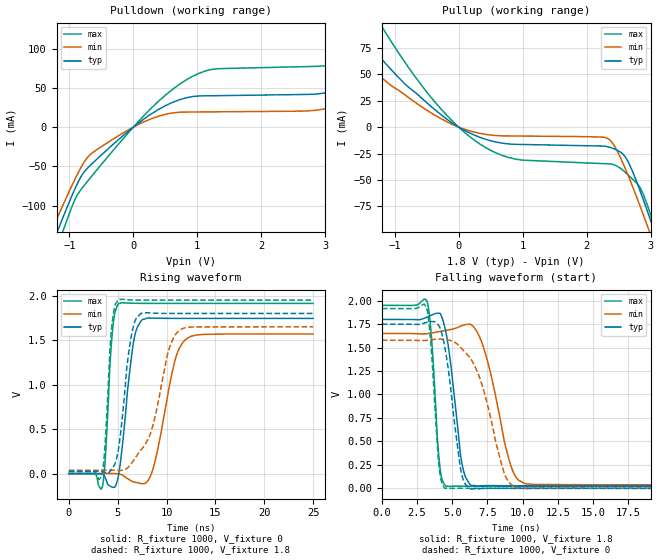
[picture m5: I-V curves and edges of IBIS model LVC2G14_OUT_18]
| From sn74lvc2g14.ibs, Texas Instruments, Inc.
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[Model]   LVC2G14_OUT_18
Model_type  Output
Vref =   0
Rref =   1000
Cref =   30p
Vmeas =   0.9
| variable   typ   min   max
C_comp   9.80pF   6.40pF   16.42pF
| C_pullup   9.15pF   6.40pF   10.43pF
| C_pulldown   10.45pF   6.59pF   16.42pF
[Temperature Range]   40   100   -40
| Ambient temperature   25   85   -40
[Voltage range]   1.8   1.65   1.95
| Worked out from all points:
|   slope of the pulldown table from 0 to 0.27 V, typ, clamps not added: 16.6 ohm
|   slope of the pullup table from 0 to 0.27 V, typ, clamps not added: 33 ohm
|   rising waveform, R_fixture 1000, V_fixture 0: 20-80 % time 995ps typ, 1.65ns min, 567ps max; typ from 0 V to 1.74 V
|   falling waveform, R_fixture 1000, V_fixture 1.8: 20-80 % time 780ps typ, 1.38ns min, 461ps max; typ from 1.8 V to 0.027 V
|   rising waveform, R_fixture 1000, V_fixture 1.8: 20-80 % time 1.02ns typ, 2.1ns min, 565ps max; typ from 0.027 V to 1.8 V
|   falling waveform, R_fixture 1000, V_fixture 0: 20-80 % time 868ps typ, 1.68ns min, 494ps max; typ from 1.75 V to 0 V
[Pulldown]
| LVC2G14_OUT_18
|   Voltage   I(typ)   I(min)   I(max)
-5.5V     -1.024A    -932.8mA   -1.143A
-1.25V    -145.7mA   -126.9mA   -167.2mA
-1.105V   -116mA     -100.2mA   -133.6mA
-650mV    -46.91mA   -33.3mA    -62.35mA
825mV     37.35mA    19.19mA    60.06mA
3.115V    45.49mA    25.17mA    79.66mA
3.755V    64.52mA    35.93mA    102.7mA
4.19V     79.14mA    21.53mA    128.2mA
4.47V     45.47mA    21.68mA    146.2mA
4.725V    44.49mA    21.83mA    131.7mA
5.01V     44.71mA    22mA       83.05mA
11V       50.72mA    25.33mA    92.94mA
[Pullup]
| LVC2G14_OUT_18
|   Voltage   I(typ)   I(min)   I(max)
-5.5V     449.7mA    254mA      638.5mA
-2.225V   143.3mA    107.6mA    207.3mA
-1.755V   105.1mA    78.04mA    153.5mA
-1.195V   63.95mA    46.44mA    94.81mA
-375mV    16.75mA    11.48mA    24.15mA
420mV     -11.47mA   -6.842mA   -19.31mA
2.34V     -18.76mA   -11.2mA    -34.79mA
2.645V    -32.43mA   -45.25mA   -45.19mA
2.84V     -61.19mA   -75.65mA   -57.82mA
2.99V     -86.8mA    -100.4mA   -81.09mA
3.08V     -102.8mA   -115.6mA   -97.77mA
11V       -1.709A    -1.61A     -1.847A
[Ramp]
| LVC2G14_OUT_18
| variable   typ   min   max
dV/dt_r   1.14/1.10E-09   1.01/1.80E-09   1.26/6.47E-10
dV/dt_f   1.10/8.47E-10   1.03/1.54E-09   1.20/5.07E-10
R_load = 1000
[Rising Waveform]
| LVC2G14_OUT_18
R_fixture =   1000
C_fixture =   0
L_fixture =   0
V_fixture =   0
V_fixture_min = 0
V_fixture_max = 0
|   Time   V(typ)   V(min)   V(max)
0s        112.7pV    7.663nV    3.037nV
3.43ns    -5.773mV   562.7uV    -148.1mV
4.45ns    -152.6mV   1.042mV    1.576V
5.115ns   -2.543mV   -3.276mV   1.911V
6.58ns    1.45V      -91.2mV    1.915V
7.51ns    1.729V     -113.8mV   1.913V
8.635ns   1.748V     59.81mV    1.913V
10.87ns   1.745V     1.273V     1.913V
11.9ns    1.744V     1.502V     1.913V
24.99ns   1.744V     1.569V     1.913V
[Falling Waveform]
| LVC2G14_OUT_18
R_fixture =   1000
C_fixture =   0
L_fixture =   0
V_fixture =   1.8
V_fixture_min = 1.65
V_fixture_max = 1.95
|   Time   V(typ)   V(min)   V(max)
0s        1.8V       1.65V      1.95V
3.225ns   1.826V     1.648V     1.988V
3.54ns    1.846V     1.656V     1.578V
4.075ns   1.867V     1.671V     293.4mV
4.54ns    1.668V     1.683V     22.36mV
5.625ns   317.2mV    1.731V     22.78mV
6.35ns    30.97mV    1.743V     21.2mV
7.295ns   27.96mV    1.464V     20.94mV
9.76ns    27.2mV     80.73mV    21.09mV
24.99ns   26.98mV    37.16mV    21.09mV
[Rising Waveform]
| LVC2G14_OUT_18
R_fixture =   1000
C_fixture =   0
L_fixture =   0
V_fixture =   1.8
V_fixture_min = 1.65
V_fixture_max = 1.95
|   Time   V(typ)   V(min)   V(max)
0s        26.95mV    37.1mV     21.07mV
3.365ns   24.61mV    37.5mV     -21.4mV
3.7ns     12.05mV    37.6mV     297.1mV
4.39ns    51.13mV    37.65mV    1.641V
5.125ns   303.9mV    35.74mV    1.958V
6.305ns   1.486V     98.9mV     1.952V
7.365ns   1.798V     262.7mV    1.95V
10.32ns   1.8V       1.421V     1.95V
11.41ns   1.8V       1.617V     1.95V
24.99ns   1.8V       1.65V      1.95V
[Falling Waveform]
| LVC2G14_OUT_18
R_fixture =   1000
C_fixture =   0
L_fixture =   0
V_fixture =   0
V_fixture_min = 0
V_fixture_max = 0
|   Time   V(typ)   V(min)   V(max)
0s        1.749V     1.578V     1.916V
3.185ns   1.769V     1.577V     1.914V
3.5ns     1.776V     1.584V     1.504V
4.035ns   1.734V     1.591V     267.6mV
4.485ns   1.492V     1.587V     -778.4uV
5.58ns    212.4mV    1.504V     1.161mV
6.295ns   -4.956mV   1.385V     16.32uV
8.685ns   195.3uV    162.8mV    5.239uV
9.5ns     77.15uV    11.32mV    17.17uV
24.99ns   22.53uV    45.99uV    14.09uV
